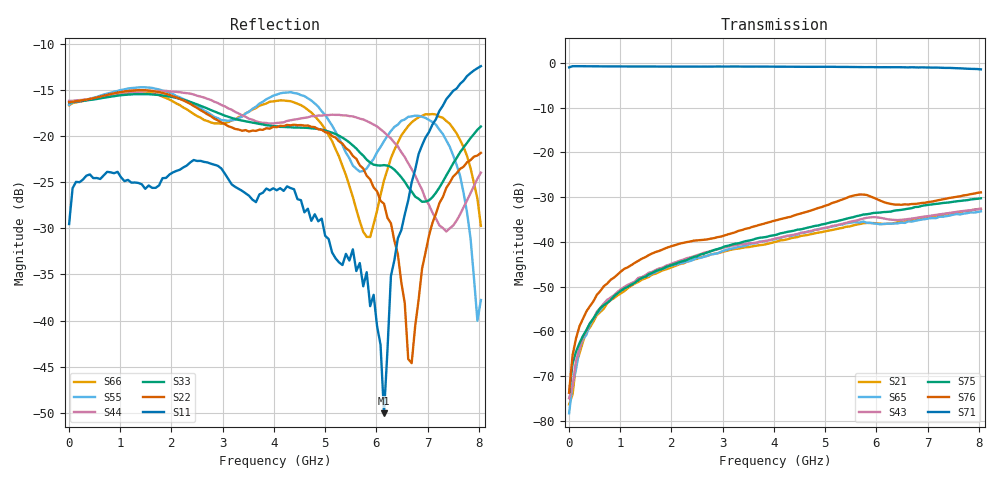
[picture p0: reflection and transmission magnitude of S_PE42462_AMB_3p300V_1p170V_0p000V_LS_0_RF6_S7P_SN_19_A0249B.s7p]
! Device ID: PE42462
! File Path: z:\PE42462\DataSheet S-parameter-6T\AMB\3p300\LS_0_RF6\PE42462_AMB_3p300V_1p170V_0p000V_LS_0_RF6_S7P_SN_19_A0249B.s7p
! Serial: 19
! Lot: A0249B
! Temp: AMB
! VDD: 3.300
! VSS: 0.000
! Control_Hi: 1.170
! Control_Lo: 0.000
! Logic State: LS_0_RF6
! Port 1:
! Port 2:
! Port 3:
! Port 4:
! Port 5:
! Port 6:
! Port 7:
! ThroughPath:1-7
! IDD: 0.0001079883
! ISS/IDD2: -4.29e-008
! IDMM3/IDD3: -1.141e-007
! Comment:
#  Hz  S  RI  R  50
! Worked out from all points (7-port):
!   120 points, 10 MHz to 8.037 GHz, reference 50 ohm
!   strongest paths, dB at 10 MHz, 2.034 GHz, 4.057 GHz, 6.08 GHz, 8.037 GHz:
!     S71: -1.0, -0.8, -0.8, -1.0, -1.4
!     S76: -73.7, -40.9, -35.2, -30.8, -28.9
!     S75: -73.8, -45.1, -38.4, -33.4, -30.3
!     S43: -75.0, -44.8, -39.2, -34.6, -32.6
!     S65: -78.3, -45.2, -39.3, -36.1, -33.2
!     S21: -76.4, -45.6, -39.9, -35.9, -32.6
!   lowest |S11| = -50.1 dB at 6.148 GHz (marker M1), VSWR 1.01, Z = 50 + j0.311 ohm
!   |S11| at or under -10 dB: start of sweep to end of sweep
